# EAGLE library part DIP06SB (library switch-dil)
DIL/CODE SWITCH
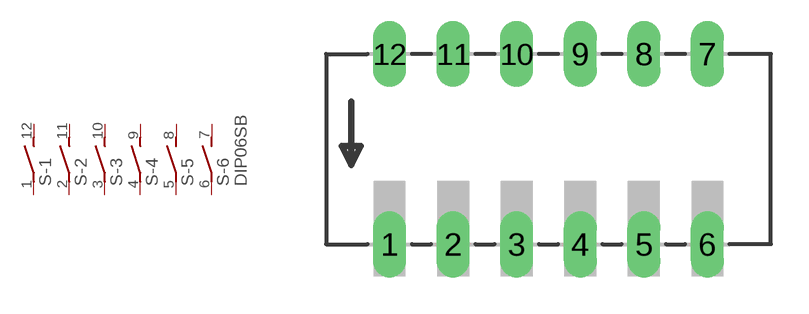
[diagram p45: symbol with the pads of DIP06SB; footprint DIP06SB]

Designator prefix S; gates -1=S -2=S -3=S -4=S -5=S -6=S+V

## DIP06SB (OC_FARNELL: unknown; OC_NEWARK: unknown)  [DIP06SB]
1  -1:1  pas
2  -2:1  pas
3  -3:1  pas
4  -4:1  pas
5  -5:1  pas
6  -6:1  pas
7  -6:2  pas
8  -5:2  pas
9  -4:2  pas
10  -3:2  pas
11  -2:2  pas
12  -1:2  pas

## Footprint DIP06SB (pad centres in mm)
DIL/CODE SWITCH
drill 0.813 long: 1 -6.35,-3.81; 2 -3.81,-3.81; 3 -1.27,-3.81; 4 1.27,-3.81; 5 3.81,-3.81; 6 6.35,-3.81; 7 6.35,3.81; 8 3.81,3.81; 9 1.27,3.81; 10 -1.27,3.81; 11 -3.81,3.81; 12 -6.35,3.81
